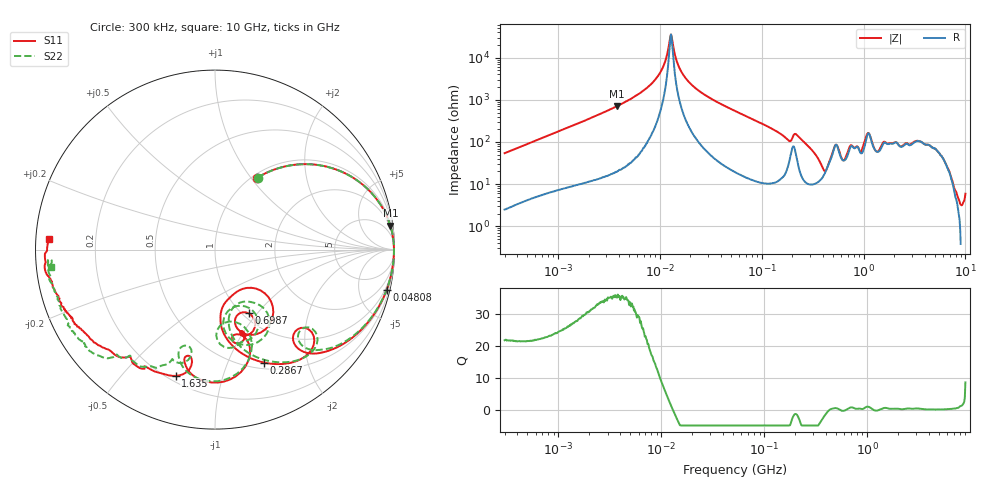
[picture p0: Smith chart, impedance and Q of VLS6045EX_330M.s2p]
! S-Parameter Data Generated by TDK Corporation
! Copyright(C) 2019 TDK Corporation.
! All Rights Reserved.
! TDK P/N: VLS6045EX-330M (Inductor)
! Property: L=33uH at 100kHz
! Size(LxWxT): 6x6x4.5mm
! Model Type: s2p (Touchstone File Format Version 1.0)
! Frequency: DC=Yes Start=0.3MHz Stop=10000MHz 802points Log-sweep
! Model Generated on May 10, 2019
! Port Assignments:
!  1 ---@@@--- 2
! Applicable Conditions:
!  Temperature = 25 degC
!  DC Bias Current = 0 A
!  Small Signal Operation
! Terms and conditions regarding TDK Simulation Models
! (1)This simulation model is being provided solely for informational purposes. Please refer to the specifications of the products in terms of detailed characteristics of such products.
! (2)In no event shall TDK Corporation of any of its subsidiaries be liable for any loss or damage arising, directly or indirectly,
!  From any information contained in this simulation model, including, but not limited to loss or damages arising from any inaccuracies, omissions or errors in connection with such information.
! (3)Any and all copyrights on this simulation model are owned by TDK Corporation.
!  Duplication or redistribution of this simulation model without prior written permission from TDK Corporation is prohibited.
! (4)This simulation model is subject to any modification or change without any prior notice.
! (5)Neither TDK Corporation nor any of its subsidiaries shall make any warranty, express or implied,
!  Including but not limited to the correctness, implied warranties of merchantability and fitness for a particular purpose with respect to this simulation models.
! (6)The use of this simulation model shall be deemed to have consented to the terms and conditions hereof.
# Hz S MA R 50
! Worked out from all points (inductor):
!   801 points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, 300 kHz to 10 GHz, reference 50 ohm
!   read as one part in series: L = 28.5 uH near 318.3 kHz
!   highest Q = 35.6 at 3.777 MHz (marker M1), where L = 29.5 uH
!   self-resonance near 12.73 MHz
!   S11 on the Smith chart (normalised r, x): 300 kHz: 1.05, +1.08; 48.08 MHz: 0.67, -8.61; 286.7 MHz: 0.57, -1.36; 698.7 MHz: 1.07, -0.90; 1.635 GHz: 0.23, -0.71; 10 GHz: 0.04, +0.03
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300000  0.4658 59.5  0.8636 -27.9  0.8638 -27.9  0.4654 59.4
1713600  0.9387 18.1  0.314 -69.9  0.3142 -69.9  0.9388 18.1
3777497  0.9861 7.7  0.1407 -80.7  0.1406 -80.6  0.9862 7.8
9671944  0.9969 0.6  0.02653 -83.6  0.02655 -83.6  0.9971 0.7
1.289893e7  0.9971 -1.2  0.002811 -0.5  0.002805 -0.3  0.9973 -1.1
1.49005e7  0.9969 -2.1  0.01342 75.4  0.01343 75.3  0.9971 -2.0
1.877128e7  0.9961 -3.7  0.03481 81.1  0.03482 81.1  0.9963 -3.5
4.807744e7  0.9824 -13.2  0.1539 74.9  0.1539 74.9  0.9826 -12.8
5.477226e7  0.9777 -15.2  0.1778 73.1  0.1778 73.1  0.978 -14.7
2.195581e8  0.7724 -45.5  0.4567 29.8  0.4566 29.8  0.7802 -44.2
2.867479e8  0.6856 -66.6  0.6591 18.9  0.659 18.9  0.6904 -64.1
3.126428e8  0.6319 -72.3  0.7028 12.7  0.7027 12.7  0.638 -69.2
4.627802e8  0.2686 -66.8  0.7112 -28.4  0.7111 -28.5  0.3475 -56.7
5.663179e8  0.5278 -61.1  0.5176 -23.3  0.5175 -23.3  0.5595 -71.9
6.987102e8  0.4008 -62.2  0.6107 -50.7  0.6105 -50.7  0.3582 -62.0
9.789263e8  0.4935 -73.6  0.5237 -71.2  0.5234 -71.2  0.4175 -74.6
1.149233e9  0.7411 -88.8  0.2587 -63.1  0.2584 -63.2  0.7335 -88.8
1.387199e9  0.6179 -105.3  0.4072 -73.2  0.4067 -73.2  0.577 -109.2
1.635219e9  0.7372 -107.4  0.2704 -90.4  0.2697 -90.4  0.6633 -109.3
1.767019e9  0.7528 -114.1  0.2633 -94.0  0.2626 -93.9  0.6614 -111.5
3.556288e9  0.8542 -145.4  0.09148 -124.1  0.09239 -124.1  0.8905 -139.5
1e10  0.926 176.2  0.04627 -166.7  0.04587 -166.6  0.918 -174.0
